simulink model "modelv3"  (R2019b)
settings: Solver=VariableStepAuto  StartTime=0.0  StopTime=500  RelTol=1e-3

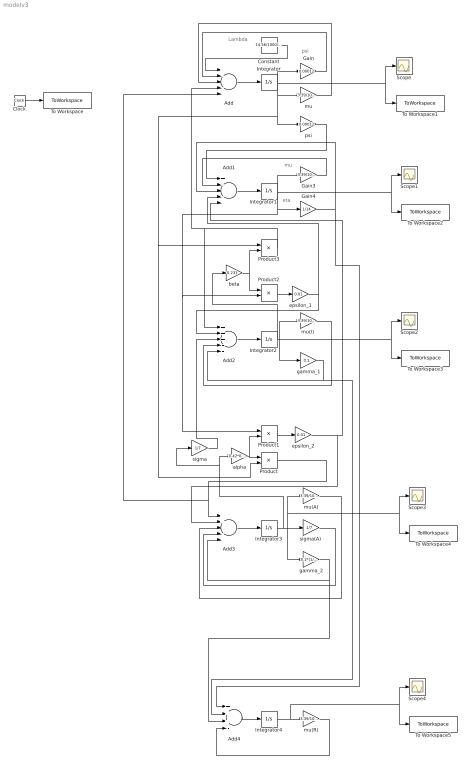
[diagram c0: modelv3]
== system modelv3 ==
  note: eta
  note: psi
  note: Lambda
  note: mu
  Add : Sum  Inputs=+----
  Add1 : Sum  Inputs=+----
  Add2 : Sum  Inputs=+++--
  Add3 : Sum  Inputs=++---
  Add4 : Sum  Inputs=+++-
  Clock : Clock
  Constant : Constant  Value=14.56/1000/352
  Gain : Gain  Gain=0.00012
  Gain3 : Gain  Gain=3.39/1000/352
  Gain4 : Gain  Gain=1/14
  Integrator : Integrator  InitialCondition=0.989961912
  Integrator1 : Integrator
  Integrator2 : Integrator  InitialCondition=0.0000707717
  Integrator3 : Integrator  InitialCondition=0.0000145165
  Integrator4 : Integrator  InitialCondition=0.0099528
  Product{,1..3} (4 alike) : Product
  Scope{,1..4} (5 alike) : Scope
  To Workspace : ToWorkspace  VariableName=t  SaveFormat=Timeseries  SampleTime=-1
  To Workspace1 : ToWorkspace  VariableName=S  SaveFormat=Timeseries  SampleTime=-1
  To Workspace2 : ToWorkspace  VariableName=V  SaveFormat=Timeseries  SampleTime=-1
  To Workspace3 : ToWorkspace  VariableName=I  SaveFormat=Timeseries  SampleTime=-1
  To Workspace4 : ToWorkspace  VariableName=A  SaveFormat=Timeseries  SampleTime=-1
  To Workspace5 : ToWorkspace  VariableName=R  SaveFormat=Timeseries  SampleTime=-1
  alpha : Gain  Gain=0.42*0.233
  beta : Gain  Gain=0.233
  epsilon_1 : Gain  Gain=0.01
  epsilon_2 : Gain  Gain=0.01
  gamma_1 : Gain  Gain=0.1
  gamma_2 : Gain  Gain=0.2*(1/7)
  mu : Gain  Gain=3.39/1000/352
  mu(A) : Gain  Gain=3.39/1000/352
  "mu(I) " : Gain  Gain=3.39/1000/352
  mu(R) : Gain  Gain=3.39/1000/352
  psi : Gain  Gain=0.00012
  sigma : Gain  Gain=1/7
  "sigma(A) " : Gain  Gain=1/7
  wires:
  Integrator/1 -> Product3/1, Product/2, psi/1, mu/1, To Workspace1/1, Scope/1, Gain/1
  Constant/1 -> Add/1
  Gain/1 -> Add/2
  mu/1 -> Add/3
  Add/1 -> Integrator/1
  Add1/1 -> Integrator1/1
  psi/1 -> Add1/1
  Gain3/1 -> Add1/2
  Gain4/1 -> Add4/1, Add1/3
  Add2/1 -> Integrator2/1
  "mu(I) "/1 -> Add2/4
  Add3/1 -> Integrator3/1
  gamma_2/1 -> Add4/3, Add3/5
  "sigma(A) "/1 -> Add3/4
  mu(A)/1 -> Add3/3
  Add4/1 -> Integrator4/1
  mu(R)/1 -> Add4/4
  gamma_1/1 -> Add4/2, Add2/5
  Product/1 -> Add/5, Add3/1
  alpha/1 -> Product1/2, Product/1
  Product1/1 -> epsilon_2/1
  epsilon_2/1 -> Add1/5, Add3/2
  sigma/1 -> Add2/3
  beta/1 -> Product3/2, Product2/1
  Product2/1 -> epsilon_1/1
  epsilon_1/1 -> Add1/4, Add2/2
  Product3/1 -> Add2/1, Add/4
  Integrator1/1 -> To Workspace2/1, Scope1/1, Product2/2, Product1/1, Gain4/1, Gain3/1
  Integrator2/1 -> beta/1, Scope2/1, To Workspace3/1, "mu(I) "/1, gamma_1/1
  Integrator3/1 -> sigma/1, alpha/1, To Workspace4/1, Scope3/1, mu(A)/1, "sigma(A) "/1, gamma_2/1
  Integrator4/1 -> To Workspace5/1, Scope4/1, mu(R)/1
  Clock/1 -> To Workspace/1
